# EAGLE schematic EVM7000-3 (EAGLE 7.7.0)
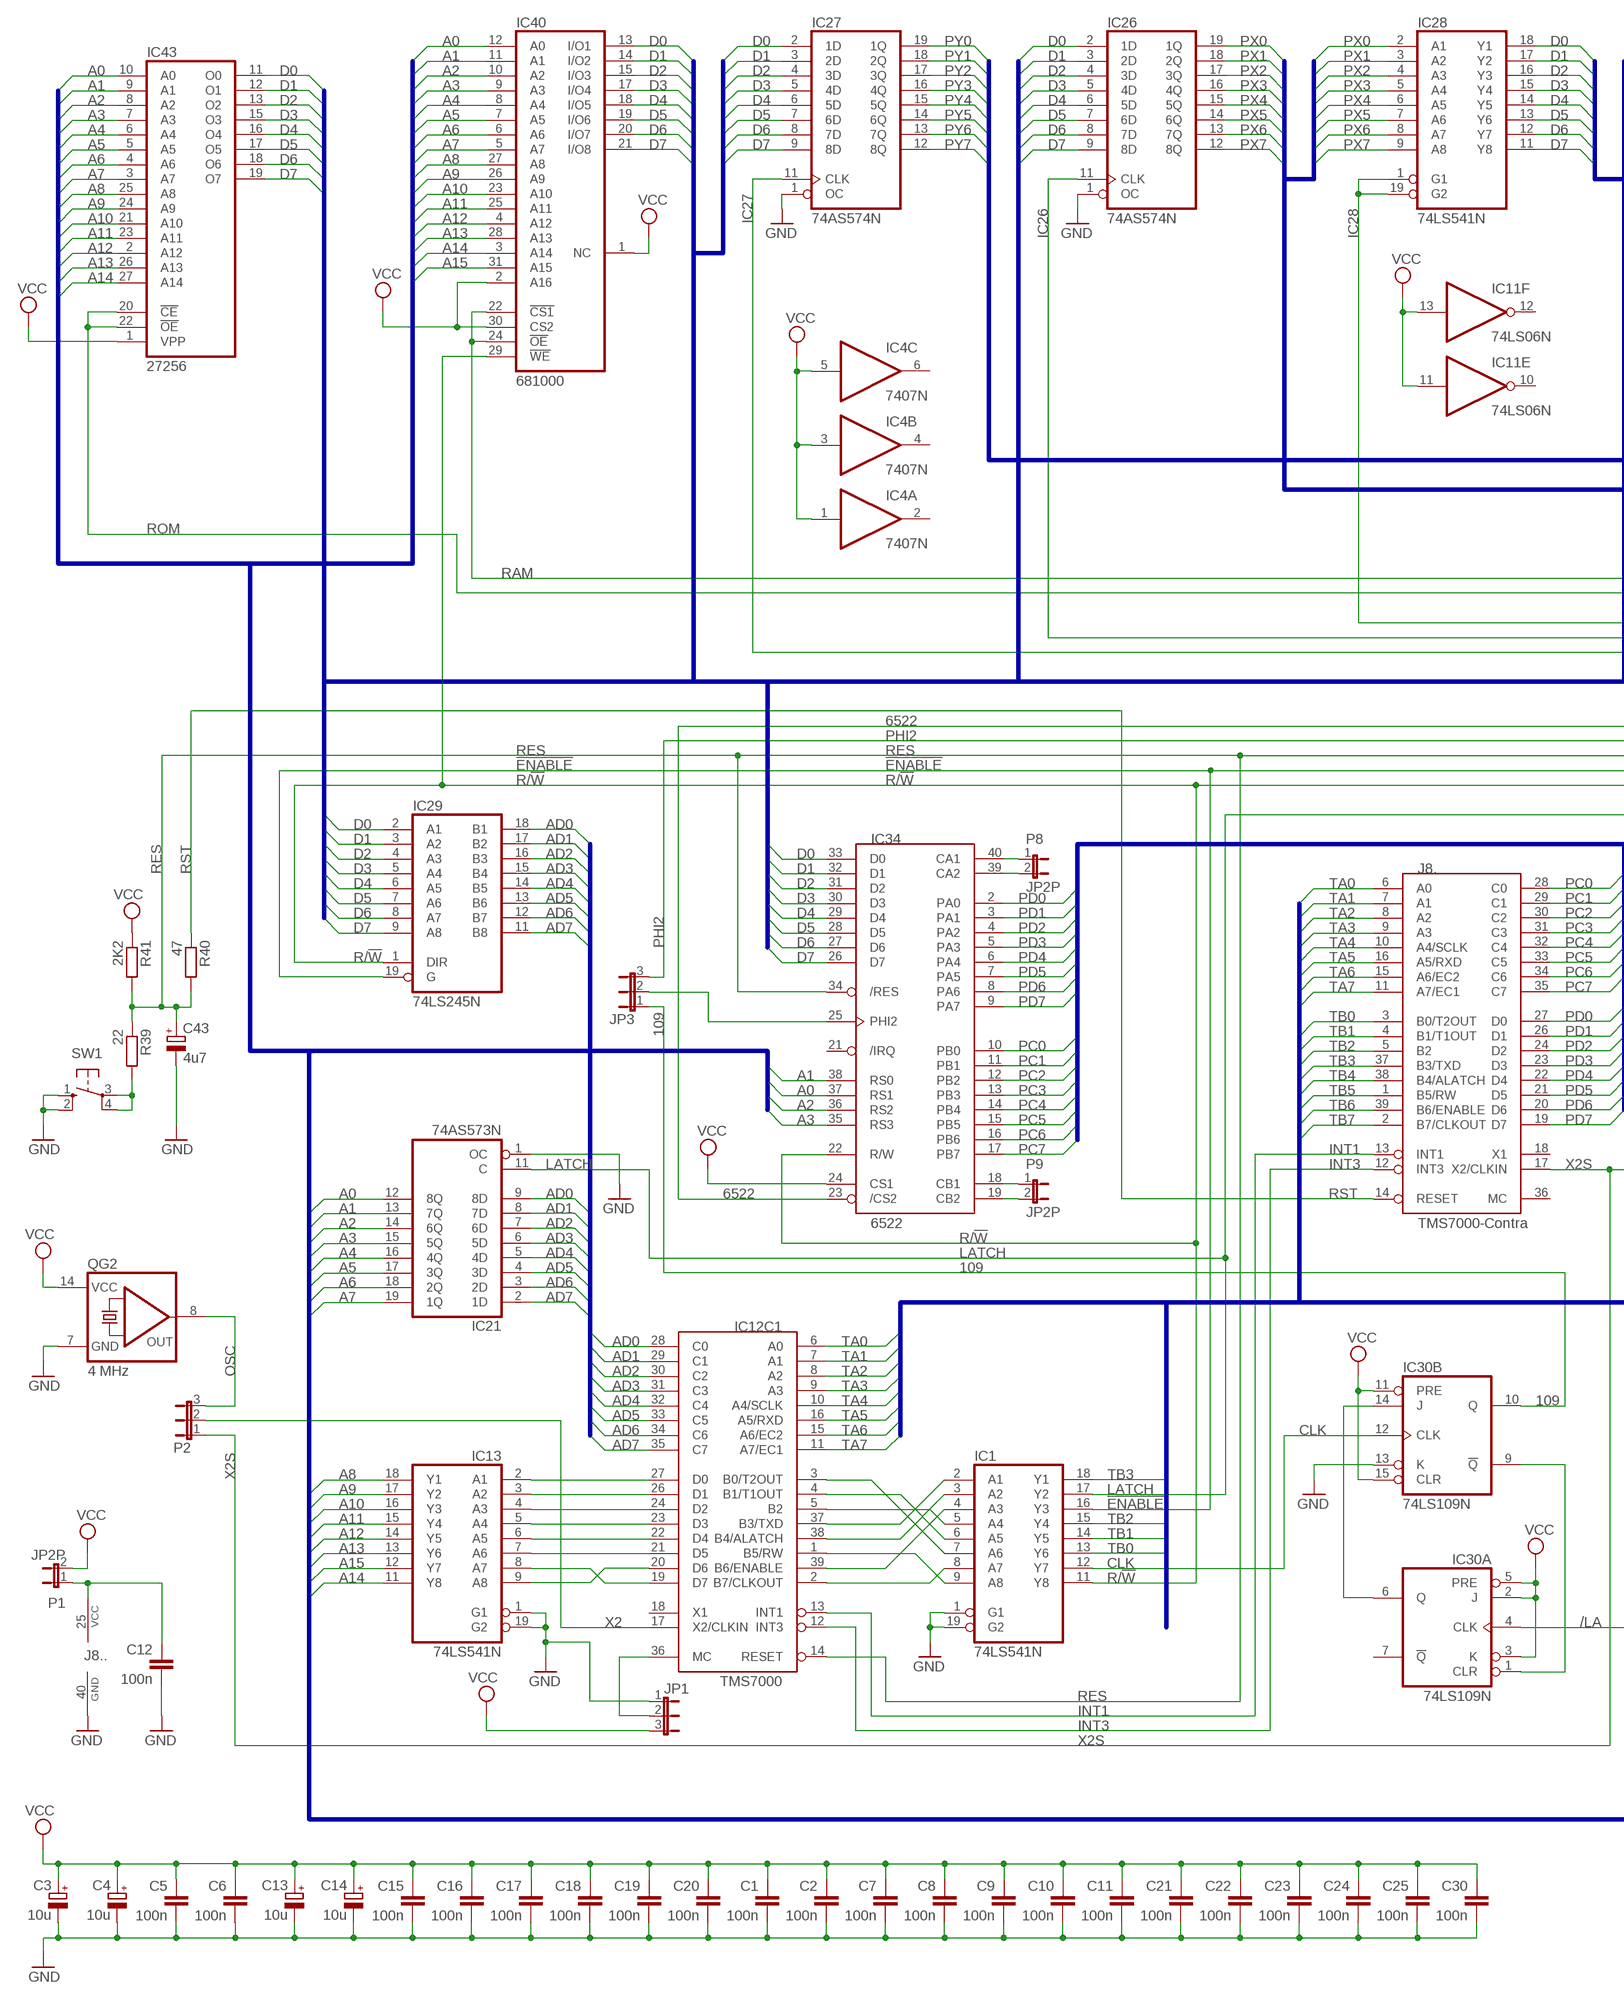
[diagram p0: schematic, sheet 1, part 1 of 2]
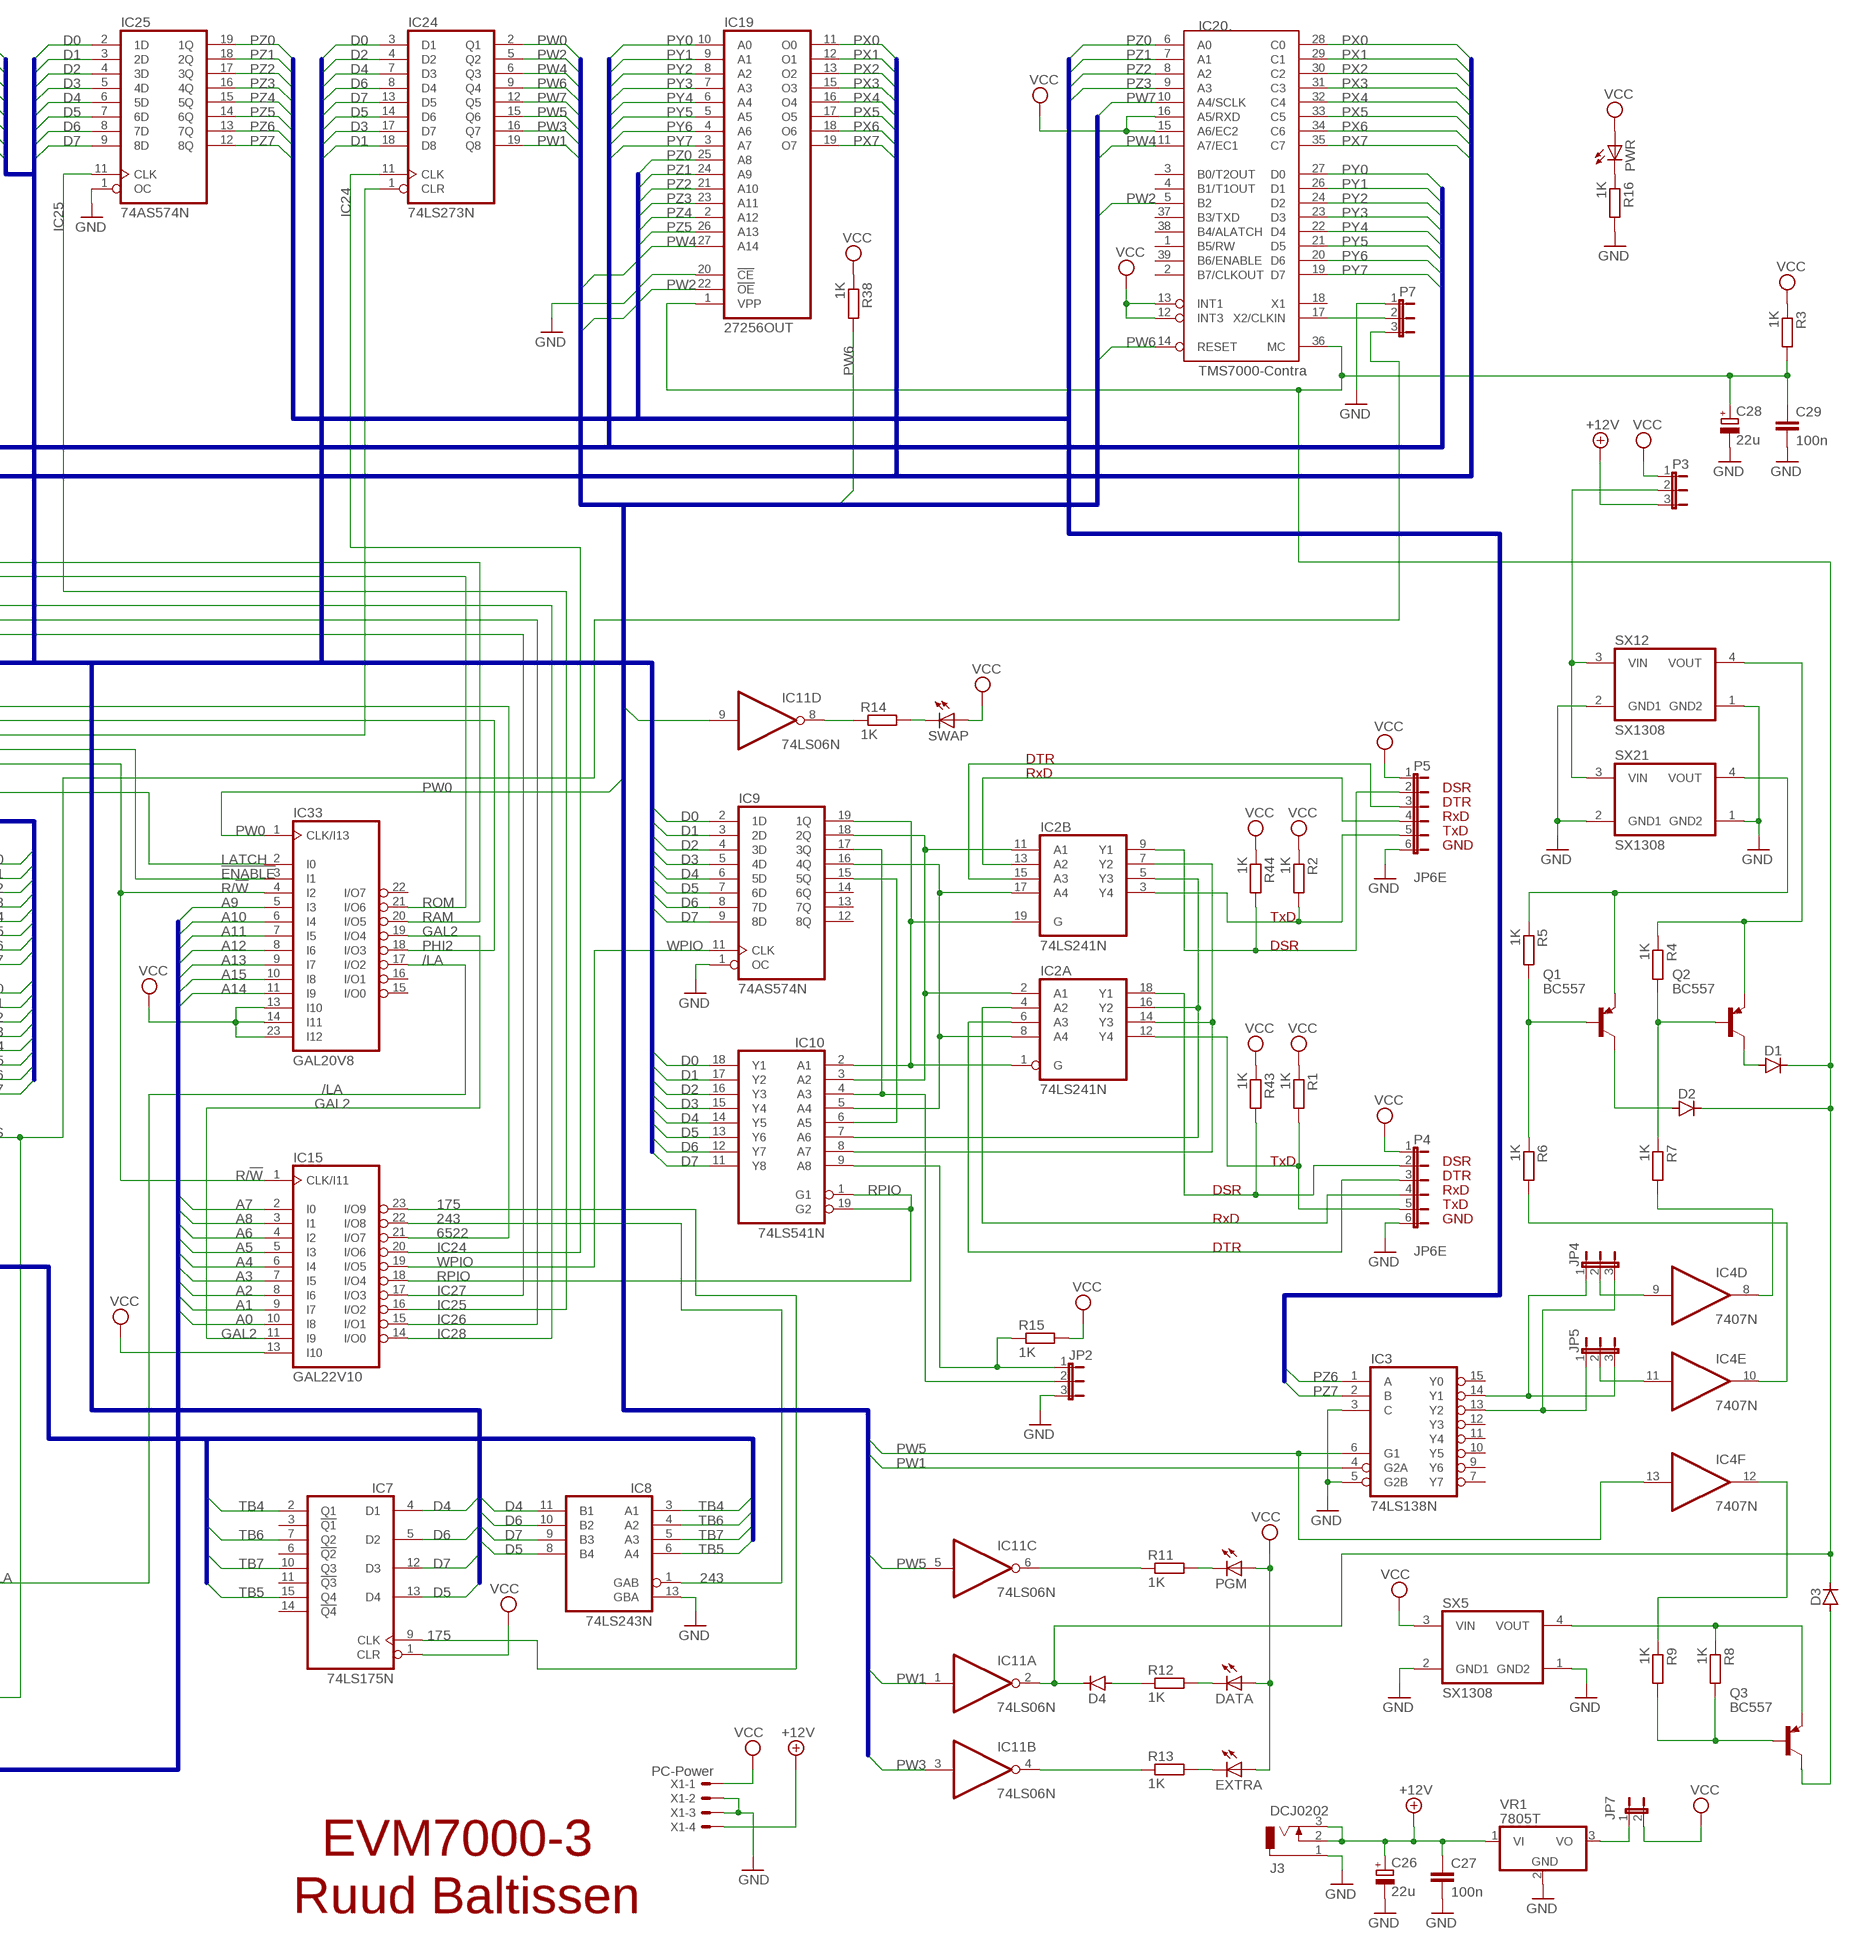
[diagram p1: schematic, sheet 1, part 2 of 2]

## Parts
C1  100n  C-EU050-024X044  [C050-024X044]
C2  100n  C-EU050-024X044  [C050-024X044]
C3  10u  CPOL-EUE5-4  [E5-4]
C4  10u  CPOL-EUE5-4  [E5-4]
C5  100n  C-EU050-024X044  [C050-024X044]
C6  100n  C-EU050-024X044  [C050-024X044]
C7  100n  C-EU050-024X044  [C050-024X044]
C8  100n  C-EU050-024X044  [C050-024X044]
C9  100n  C-EU050-024X044  [C050-024X044]
C10  100n  C-EU050-024X044  [C050-024X044]
C11  100n  C-EU050-024X044  [C050-024X044]
C12  100n  C-EU050-024X044  [C050-024X044]
C13  10u  CPOL-EUE5-4  [E5-4]
C14  10u  CPOL-EUE5-4  [E5-4]
C15  100n  C-EU050-024X044  [C050-024X044]
C16  100n  C-EU050-024X044  [C050-024X044]
C17  100n  C-EU050-024X044  [C050-024X044]
C18  100n  C-EU050-024X044  [C050-024X044]
C19  100n  C-EU050-024X044  [C050-024X044]
C20  100n  C-EU050-024X044  [C050-024X044]
C21  100n  C-EU050-024X044  [C050-024X044]
C22  100n  C-EU050-024X044  [C050-024X044]
C23  100n  C-EU050-024X044  [C050-024X044]
C24  100n  C-EU050-024X044  [C050-024X044]
C25  100n  C-EU050-024X044  [C050-024X044]
C26  22u  CPOL-EUE2,5-6E  [E2,5-6E]
C27  100n  C-EU050-024X044  [C050-024X044]
C28  22u  CPOL-EUE2,5-6E  [E2,5-6E]
C29  100n  C-EU050-024X044  [C050-024X044]
C30  100n  C-EU050-024X044  [C050-024X044]
C43  4u7  CPOL-EUE5-4  [E5-4]
D1  DIODE-S2  [0207/2V]
D2  DIODE-S2  [0207/2V]
D3  DIODE-S2  [0207/2V]
D4  DIODE-S2  [0207/2V]
DATA  TLLY4400  [LED3MM]
EXTRA  TLLY4400  [LED3MM]
IC1  74LS541N  [DIL20]
IC2  74LS241N  [DIL20]
IC3  74LS138N  [DIL16]
IC4  7407N  [DIL14]
IC7  74LS175N  [DIL16]
IC8  74LS243N  [DIL14]
IC9  74AS574N  [DIL20]
IC10  74LS541N  [DIL20]
IC11  74LS06N  [DIL14]
IC12  TMS7000  [DIL40]
IC13  74LS541N  [DIL20]
IC15  GAL22V10  [DIL24-3]
IC19  27256OUT  [DIL28]
IC20  TMS7000-Contra  TMS7000CON  [DIL40]
IC21  74AS573N  [DIL20]
IC24  74LS273N  74273N  [DIL20]
IC25  74AS574N  [DIL20]
IC26  74AS574N  [DIL20]
IC27  74AS574N  [DIL20]
IC28  74LS541N  [DIL20]
IC29  74LS245N  [DIL20]
IC30  74LS109N  [DIL16]
IC33  GAL20V8  [DIL24-3]
IC34  6522  [DIP40]
IC40  681000  [DIL32-6]
IC43  27256  [DIL28]
J3  DCJ0202  [DCJ0202]
J8  TMS7000-Contra  TMS7000CON  [DIL40]
JP1  JP2E  [JP2]
JP2  JP2E  [JP2]
JP3  JP2E  [JP2]
JP4  JP2E  [JP2]
JP5  JP2E  [JP2]
JP7  JP2P  [JP2P]
P1  JP2P  [JP2P]
P2  JP2E  [JP2]
P3  JP2E  [JP2]
P4  JP6E  [JP6E]
P5  JP6E  [JP6E]
P7  JP2E  [JP2]
P8  JP2P  [JP2P]
P9  JP2P  [JP2P]
PGM  TLLY4400  [LED3MM]
PWR  TLLY4400  [LED3MM]
Q1  BC557  [TO92-EBC]
Q2  BC557  [TO92-EBC]
Q3  BC557  [TO92-EBC]
QG2  4 MHz  QG5860  [DIL14S]
R1  1K  R-EU_0204/2V  [0204V]
R2  1K  R-EU_0204/2V  [0204V]
R3  1K  R-EU_0204/2V  [0204V]
R4  1K  R-EU_0204/2V  [0204V]
R5  1K  R-EU_0204/2V  [0204V]
R6  1K  R-EU_0204/2V  [0204V]
R7  1K  R-EU_0204/2V  [0204V]
R8  1K  R-EU_0204/2V  [0204V]
R9  1K  R-EU_0204/2V  [0204V]
R11  1K  R-EU_0204/2V  [0204V]
R12  1K  R-EU_0204/2V  [0204V]
R13  1K  R-EU_0204/2V  [0204V]
R14  1K  R-EU_0204/2V  [0204V]
R15  1K  R-EU_0204/2V  [0204V]
R16  1K  R-EU_0204/2V  [0204V]
R38  1K  R-EU_0204/2V  [0204V]
R39  22  R-EU_0204/2V  [0204V]
R40  47  R-EU_0204/2V  [0204V]
R41  2K2  R-EU_0204/2V  [0204V]
R43  1K  R-EU_0204/2V  [0204V]
R44  1K  R-EU_0204/2V  [0204V]
SW1  10-XX  [B3F-10XX]
SWAP  TLLY4400  [LED3MM]
SX5  SX1308  [SX1308]
SX12  SX1308  [SX1308]
SX21  SX1308  [SX1308]
VR1  7805T  [TO220H]
X1  PC-Power  22-23-2041  [22-23-2041]

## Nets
109: IC30.10(B:Q) JP3.1
175: IC7.9(CLK) IC15.23(I/O9)
243: IC8.1(GAB) IC15.22(I/O8)
6522: IC15.21(I/O7) IC34.23(/CS2)
!ENABLE: IC1.16(Y3) IC29.19(G) IC33.3(I1)
+12V: C26.+ C27.1 J3.2 J3.3 P3.3 VR1.1(VI) X1.4
/LA: IC30.4(A:CLK) IC33.17(I/O2)
A0: IC15.10(I8) IC21.12(8Q) IC34.37(RS1) IC40.12(A0) IC43.10(A0)
A1: IC15.9(I7) IC21.13(7Q) IC34.38(RS0) IC40.11(A1) IC43.9(A1)
A2: IC15.8(I6) IC21.14(6Q) IC34.36(RS2) IC40.10(A2) IC43.8(A2)
A3: IC15.7(I5) IC21.15(5Q) IC34.35(RS3) IC40.9(A3) IC43.7(A3)
A4: IC15.6(I4) IC21.16(4Q) IC40.8(A4) IC43.6(A4)
A5: IC15.5(I3) IC21.17(3Q) IC40.7(A5) IC43.5(A5)
A6: IC15.4(I2) IC21.18(2Q) IC40.6(A6) IC43.4(A6)
A7: IC15.2(I0) IC21.19(1Q) IC40.5(A7) IC43.3(A7)
A8: IC13.18(Y1) IC15.3(I1) IC40.27(A8) IC43.25(A8)
A9: IC13.17(Y2) IC33.5(I3) IC40.26(A9) IC43.24(A9)
A10: IC13.16(Y3) IC33.6(I4) IC40.23(A10) IC43.21(A10)
A11: IC13.15(Y4) IC33.7(I5) IC40.25(A11) IC43.23(A11)
A12: IC13.14(Y5) IC33.8(I6) IC40.4(A12) IC43.2(A12)
A13: IC13.13(Y6) IC33.9(I7) IC40.28(A13) IC43.26(A13)
A14: IC13.11(Y8) IC33.11(I9) IC40.3(A14) IC43.27(A14)
A15: IC13.12(Y7) IC33.10(I8) IC40.31(A15)
AD0: IC12.28(C1:C0) IC21.9(8D) IC29.18(B1)
AD1: IC12.29(C1:C1) IC21.8(7D) IC29.17(B2)
AD2: IC12.30(C1:C2) IC21.7(6D) IC29.16(B3)
AD3: IC12.31(C1:C3) IC21.6(5D) IC29.15(B4)
AD4: IC12.32(C1:C4) IC21.5(4D) IC29.14(B5)
AD5: IC12.33(C1:C5) IC21.4(3D) IC29.13(B6)
AD6: IC12.34(C1:C6) IC21.3(2D) IC29.12(B7)
AD7: IC12.35(C1:C7) IC21.2(1D) IC29.11(B8)
CLK: IC1.12(Y7) IC30.12(B:CLK)
D0: IC9.2(1D) IC10.18(Y1) IC24.3(D1) IC25.2(1D) IC26.2(1D) IC27.2(1D) IC28.18(Y1) IC29.2(A1) IC34.33(D0) IC40.13(I/O1) IC43.11(O0)
D1: IC9.3(2D) IC10.17(Y2) IC24.18(D8) IC25.3(2D) IC26.3(2D) IC27.3(2D) IC28.17(Y2) IC29.3(A2) IC34.32(D1) IC40.14(I/O2) IC43.12(O1)
D2: IC9.4(3D) IC10.16(Y3) IC24.4(D2) IC25.4(3D) IC26.4(3D) IC27.4(3D) IC28.16(Y3) IC29.4(A3) IC34.31(D2) IC40.15(I/O3) IC43.13(O2)
D3: IC9.5(4D) IC10.15(Y4) IC24.17(D7) IC25.5(4D) IC26.5(4D) IC27.5(4D) IC28.15(Y4) IC29.5(A4) IC34.30(D3) IC40.17(I/O4) IC43.15(O3)
D4: IC7.4(D1) IC8.11(B1) IC9.6(5D) IC10.14(Y5) IC24.7(D3) IC25.6(5D) IC26.6(5D) IC27.6(5D) IC28.14(Y5) IC29.6(A5) IC34.29(D4) IC40.18(I/O5) IC43.16(O4)
D5: IC7.13(D4) IC8.8(B4) IC9.7(6D) IC10.13(Y6) IC24.14(D6) IC25.7(6D) IC26.7(6D) IC27.7(6D) IC28.13(Y6) IC29.7(A6) IC34.28(D5) IC40.19(I/O6) IC43.17(O5)
D6: IC7.5(D2) IC8.10(B2) IC9.8(7D) IC10.12(Y7) IC24.8(D4) IC25.8(7D) IC26.8(7D) IC27.8(7D) IC28.12(Y7) IC29.8(A7) IC34.27(D6) IC40.20(I/O7) IC43.18(O6)
D7: IC7.12(D3) IC8.9(B3) IC9.9(8D) IC10.11(Y8) IC24.13(D5) IC25.9(8D) IC26.9(8D) IC27.9(8D) IC28.11(Y8) IC29.9(A8) IC34.26(D7) IC40.21(I/O8) IC43.19(O7)
DSR1: IC2.9(B:Y1) P5.2 R44.2
DSR2: IC2.18(A:Y1) P4.2 R43.2
DTR1: IC2.15(B:A3) P5.3
DTR2: IC2.6(A:A3) P4.3
GAL2: IC15.11(I9) IC33.19(I/O4)
GND: C1.2 C2.2 C3.- C4.- C5.2 C6.2 C7.2 C8.2 C9.2 C10.2 C11.2 C12.2 C13.- C14.- C15.2 C16.2 C17.2 C18.2 C19.2 C20.2 C21.2 C22.2 C23.2 C24.2 C25.2 C26.- C27.2 C28.- C29.2 C30.2 C43.- IC1.1(G1) IC1.19(G2) IC3.3(C) IC3.5(G2B) IC8.13(GBA) IC9.1(OC) IC13.1(G1) IC13.19(G2) IC19.20(!CE) IC21.1(OC) IC25.1(OC) IC26.1(OC) IC27.1(OC) IC30.13(B:K) J3.1 J8.40(..:GND) JP1.1 JP2.3 P4.6 P5.6 P7.1 QG2.7(GND) R16.2 SW1.1(S) SW1.2(S1) SX5.1(GND2) SX5.2(GND1) SX12.1(GND2) SX12.2(GND1) SX21.1(GND2) SX21.2(GND1) VR1.2(GND) X1.2 X1.3
IC24: IC15.20(I/O6) IC24.11(CLK)
IC25: IC15.16(I/O2) IC25.11(CLK)
IC26: IC15.15(I/O1) IC26.11(CLK)
IC27: IC15.17(I/O3) IC27.11(CLK)
IC28: IC15.14(I/O0) IC28.1(G1) IC28.19(G2)
INT1: IC12.13(C1:INT1) J8.13(.:INT1)
INT3: IC12.12(C1:INT3) J8.12(.:INT3)
LATCH: IC1.17(Y2) IC21.11(C) IC33.2(I0)
N$1: IC1.9(A8) IC12.1(C1:B5/RW)
N$2: IC1.8(A7) IC12.2(C1:B7/CLKOUT)
N$3: IC1.7(A6) IC12.3(C1:B0/T2OUT)
N$4: R39.2 SW1.3(P) SW1.4(P1)
N$5: IC1.6(A5) IC12.4(C1:B1/T1OUT)
N$6: IC12.19(C1:D7) IC13.8(A7)
N$7: IC12.20(C1:D6) IC13.9(A8)
N$8: IC1.5(A4) IC12.5(C1:B2)
N$9: IC1.4(A3) IC12.39(C1:B6/ENABLE)
N$10: IC12.27(C1:D0) IC13.2(A1)
N$11: IC12.26(C1:D1) IC13.3(A2)
N$12: IC12.24(C1:D2) IC13.4(A3)
N$13: IC1.3(A2) IC12.38(C1:B4/ALATCH)
N$14: C12.1 J8.25(..:VCC) P1.1
N$15: IC1.2(A1) IC12.37(C1:B3/TXD)
N$16: EXTRA.K(C) R13.2
N$17: IC12.23(C1:D3) IC13.5(A4)
N$18: IC12.22(C1:D4) IC13.6(A5)
N$19: IC12.21(C1:D5) IC13.7(A6)
N$20: IC11.4(B:O) R13.1
N$21: IC34.40(CA1) P8.1
N$22: IC34.39(CA2) P8.2
N$23: IC20.17(.:X2/CLKIN) P7.2
N$24: IC34.18(CB1) P9.1
N$25: IC34.19(CB2) P9.2
N$26: IC2.8(A:A4) IC2.17(B:A4) IC9.16(4Q) IC10.5(A4)
N$27: IC2.2(A:A1) IC2.11(B:A1) IC9.18(2Q) IC10.3(A2)
N$28: IC2.5(B:Y3) IC2.16(A:Y2) IC10.7(A6)
N$29: IC2.7(B:Y2) IC2.14(A:Y3) IC10.8(A7)
N$30: IC2.1(A:G) IC2.19(B:G) IC9.19(1Q) IC10.2(A1)
N$31: IC9.17(3Q) IC10.4(A3) JP2.2
N$32: IC9.15(5Q) IC10.6(A5)
N$33: IC4.9(D:I) JP4.2
N$34: IC4.11(E:I) JP5.2
N$36: Q1.E R5.1 SX21.4(VOUT)
N$37: Q2.E R4.1 SX12.4(VOUT)
N$38: Q1.B R5.2 R6.1
N$39: IC4.8(D:O) R7.2
N$40: Q2.B R4.2 R7.1
N$41: C28.+ C29.1 D1.2(C) D2.2(C) D3.2(C) D4.2(C) IC11.2(A:O) IC19.1(VPP) IC20.36(.:MC) R3.2
N$42: IC4.10(E:O) R6.2
N$43: Q3.B R8.2 R9.2
N$44: D1.1(A) Q2.C
N$45: IC4.12(F:O) R9.1
N$46: IC10.9(A8) JP2.1 R15.1
N$47: D2.1(A) Q1.C
N$48: D3.1(A) Q3.C
N$49: Q3.E R8.1 SX5.4(VOUT)
N$50: R14.2 SWAP.K(C)
N$51: P3.2 SX12.3(VIN) SX21.3(VIN)
N$52: IC11.8(D:O) R14.1
N$53: PWR.K(C) R16.1
N$54: IC3.14(Y1) JP4.1 JP5.3
N$55: IC3.13(Y2) JP4.3 JP5.1
N$56: PGM.K(C) R11.2
N$57: DATA.K(C) R12.2
N$58: D4.1(A) R12.1
N$59: IC12.36(C1:MC) JP1.2
N$60: IC11.6(C:O) R11.1
N$63: IC34.25(PHI2) JP3.2
N$64: IC30.6(A:Q) IC30.14(B:J)
N$65: JP7.1 VR1.3(VO)
N$66: IC30.1(A:CLR) IC30.9(B:!Q)
OSC: P2.3 QG2.8(OUT)
PC0: IC34.10(PB0) J8.28(.:C0)
PC1: IC34.11(PB1) J8.29(.:C1)
PC2: IC34.12(PB2) J8.30(.:C2)
PC3: IC34.13(PB3) J8.31(.:C3)
PC4: IC34.14(PB4) J8.32(.:C4)
PC5: IC34.15(PB5) J8.33(.:C5)
PC6: IC34.16(PB6) J8.34(.:C6)
PC7: IC34.17(PB7) J8.35(.:C7)
PD0: IC34.2(PA0) J8.27(.:D0)
PD1: IC34.3(PA1) J8.26(.:D1)
PD2: IC34.4(PA2) J8.24(.:D2)
PD3: IC34.5(PA3) J8.23(.:D3)
PD4: IC34.6(PA4) J8.22(.:D4)
PD5: IC34.7(PA5) J8.21(.:D5)
PD6: IC34.8(PA6) J8.20(.:D6)
PD7: IC34.9(PA7) J8.19(.:D7)
PHI2: IC33.18(I/O3) JP3.3
PW0: IC11.9(D:I) IC24.2(Q1) IC33.1(CLK/I13)
PW1: IC3.4(G2A) IC11.1(A:I) IC24.19(Q8)
PW2: IC19.22(!OE) IC20.5(.:B2) IC24.5(Q2)
PW3: IC11.3(B:I) IC24.16(Q7)
PW4: IC19.27(A14) IC20.11(.:A7/EC1) IC24.6(Q3)
PW5: IC3.6(G1) IC4.13(F:I) IC11.5(C:I) IC24.15(Q6)
PW6: IC20.14(.:RESET) IC24.9(Q4) R38.2
PW7: IC20.10(.:A4/SCLK) IC24.12(Q5)
PX0: IC19.11(O0) IC20.28(.:C0) IC26.19(1Q) IC28.2(A1)
PX1: IC19.12(O1) IC20.29(.:C1) IC26.18(2Q) IC28.3(A2)
PX2: IC19.13(O2) IC20.30(.:C2) IC26.17(3Q) IC28.4(A3)
PX3: IC19.15(O3) IC20.31(.:C3) IC26.16(4Q) IC28.5(A4)
PX4: IC19.16(O4) IC20.32(.:C4) IC26.15(5Q) IC28.6(A5)
PX5: IC19.17(O5) IC20.33(.:C5) IC26.14(6Q) IC28.7(A6)
PX6: IC19.18(O6) IC20.34(.:C6) IC26.13(7Q) IC28.8(A7)
PX7: IC19.19(O7) IC20.35(.:C7) IC26.12(8Q) IC28.9(A8)
PY0: IC19.10(A0) IC20.27(.:D0) IC27.19(1Q)
PY1: IC19.9(A1) IC20.26(.:D1) IC27.18(2Q)
PY2: IC19.8(A2) IC20.24(.:D2) IC27.17(3Q)
PY3: IC19.7(A3) IC20.23(.:D3) IC27.16(4Q)
PY4: IC19.6(A4) IC20.22(.:D4) IC27.15(5Q)
PY5: IC19.5(A5) IC20.21(.:D5) IC27.14(6Q)
PY6: IC19.4(A6) IC20.20(.:D6) IC27.13(7Q)
PY7: IC19.3(A7) IC20.19(.:D7) IC27.12(8Q)
PZ0: IC19.25(A8) IC20.6(.:A0) IC25.19(1Q)
PZ1: IC19.24(A9) IC20.7(.:A1) IC25.18(2Q)
PZ2: IC19.21(A10) IC20.8(.:A2) IC25.17(3Q)
PZ3: IC19.23(A11) IC20.9(.:A3) IC25.16(4Q)
PZ4: IC19.2(A12) IC25.15(5Q)
PZ5: IC19.26(A13) IC25.14(6Q)
PZ6: IC3.1(A) IC25.13(7Q)
PZ7: IC3.2(B) IC25.12(8Q)
R/!W: IC1.11(Y8) IC15.1(CLK/I11) IC29.1(DIR) IC33.4(I2) IC34.22(R/W) IC40.29(!WE)
RAM: IC33.20(I/O5) IC40.22(!CS1) IC40.24(!OE)
RES: C43.+ IC12.14(C1:RESET) IC24.1(CLR) IC34.34(/RES) R39.1 R40.2 R41.2
ROM: IC33.21(I/O6) IC43.20(!CE) IC43.22(!OE)
RPIO: IC10.1(G1) IC10.19(G2) IC15.18(I/O4)
RST: J8.14(.:RESET) R40.1
RXD1: IC2.13(B:A2) P5.4
RXD2: IC2.4(A:A2) P4.4
TA0: IC12.6(C1:A0) J8.6(.:A0)
TA1: IC12.7(C1:A1) J8.7(.:A1)
TA2: IC12.8(C1:A2) J8.8(.:A2)
TA3: IC12.9(C1:A3) J8.9(.:A3)
TA4: IC12.10(C1:A4/SCLK) J8.10(.:A4/SCLK)
TA5: IC12.16(C1:A5/RXD) J8.16(.:A5/RXD)
TA6: IC12.15(C1:A6/EC2) J8.15(.:A6/EC2)
TA7: IC12.11(C1:A7/EC1) J8.11(.:A7/EC1)
TB0: IC1.13(Y6) J8.3(.:B0/T2OUT)
TB1: IC1.14(Y5) J8.4(.:B1/T1OUT)
TB2: IC1.15(Y4) J8.5(.:B2)
TB3: IC1.18(Y1) J8.37(.:B3/TXD)
TB4: IC7.2(Q1) IC8.3(A1) J8.38(.:B4/ALATCH)
TB5: IC7.15(Q4) IC8.6(A4) J8.1(.:B5/RW)
TB6: IC7.7(Q2) IC8.4(A2) J8.39(.:B6/ENABLE)
TB7: IC7.10(Q3) IC8.5(A3) J8.2(.:B7/CLKOUT)
TXD1: IC2.3(B:Y4) P5.5 R2.2
TXD2: IC2.12(A:Y4) P4.5 R1.2
VCC: C1.1 C2.1 C3.+ C4.+ C5.1 C6.1 C7.1 C8.1 C9.1 C10.1 C11.1 C13.+ C14.+ C15.1 C16.1 C17.1 C18.1 C19.1 C20.1 C21.1 C22.1 C23.1 C24.1 C25.1 C30.1 DATA.A EXTRA.A IC4.1(A:I) IC4.3(B:I) IC4.5(C:I) IC7.1(CLR) IC11.11(E:I) IC11.13(F:I) IC15.13(I10) IC20.12(.:INT3) IC20.13(.:INT1) IC20.15(.:A6/EC2) IC20.16(.:A5/RXD) IC30.2(A:J) IC30.3(A:K) IC30.5(A:PRE) IC30.11(B:PRE) IC30.15(B:CLR) IC33.13(I10) IC33.14(I11) IC33.23(I12) IC34.24(CS1) IC40.1(NC) IC40.2(A16) IC40.30(CS2) IC43.1(VPP) JP1.3 JP7.2 P1.2 P3.1 P4.1 P5.1 PGM.A PWR.A QG2.14(VCC) R1.1 R2.1 R3.1 R15.2 R38.1 R41.1 R43.1 R44.1 SWAP.A SX5.3(VIN) X1.1
WPIO: IC9.11(CLK) IC15.19(I/O5)
X2: IC12.17(C1:X2/CLKIN) P2.2
X2S: J8.17(.:X2/CLKIN) P2.1 P7.3
Unconnected: IC3.7(Y7) IC3.9(Y6) IC3.10(Y5) IC3.11(Y4) IC3.12(Y3) IC3.15(Y0) IC4.2(A:O) IC4.4(B:O) IC4.6(C:O) IC7.3(!Q1) IC7.6(!Q2) IC7.11(!Q3) IC7.14(!Q4) IC9.12(8Q) IC9.13(7Q) IC9.14(6Q) IC11.10(E:O) IC11.12(F:O) IC12.18(C1:X1) IC20.1(.:B5/RW) IC20.2(.:B7/CLKOUT) IC20.3(.:B0/T2OUT) IC20.4(.:B1/T1OUT) IC20.18(.:X1) IC20.37(.:B3/TXD) IC20.38(.:B4/ALATCH) IC20.39(.:B6/ENABLE) IC30.7(A:!Q) IC33.15(I/O0) IC33.16(I/O1) IC33.22(I/O7) IC34.21(/IRQ) J8.18(.:X1) J8.36(.:MC)

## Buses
ADDRESSBUS:A[0..15]
DATABUS:D[0..7]
ADDA:AD[0..7]
TMS:TA[0..7],TB[0..7]
PCD:PC[0..7],PD[0..7]
PY:PY[0..7]
PX:PX[0..7]
PZ:PZ[0..7]
PW:PW[0..7]

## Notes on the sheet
- DTR
- RxD
- DSR
- DTR
- RxD
- TxD
- GND
- TxD
- DSR
- TxD | DSR
- DTR
- DSR | RxD
- TxD
- RxD | GND
- DTR
- EVM7000-3
- Ruud Baltissen

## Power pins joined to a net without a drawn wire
GND: IC1.10(GND) IC2.10(P:GND) IC3.8(GND) IC4.7(P:GND) IC7.8(GND) IC8.7(GND) IC9.10(GND) IC10.10(GND) IC11.7(P:GND) IC12.40(GND) IC13.10(GND) IC15.12(GND) IC19.14(GND) IC20.40(..:GND) IC21.10(GND) IC24.10(GND) IC25.10(GND) IC26.10(GND) IC27.10(GND) IC28.10(GND) IC29.10(GND) IC30.8(P:GND) IC33.12(GND) IC34.1(GND) IC40.16(GND) IC43.14(GND)
VCC: IC1.20(VCC) IC2.20(P:VCC) IC3.16(VCC) IC4.14(P:VCC) IC7.16(VCC) IC8.14(VCC) IC9.20(VCC) IC10.20(VCC) IC11.14(P:VCC) IC12.25(VCC) IC13.20(VCC) IC15.24(VCC) IC19.28(VCC) IC20.25(..:VCC) IC21.20(VCC) IC24.20(VCC) IC25.20(VCC) IC26.20(VCC) IC27.20(VCC) IC28.20(VCC) IC29.20(VCC) IC30.16(P:VCC) IC33.24(VCC) IC34.20(VCC) IC40.32(VCC) IC43.28(VCC)

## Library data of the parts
C1 C2 C5-C12 C15-C25 C27 C29 C30 = rcl:C-EU: CAPACITOR, European symbol
C3 C4 C13 C14 C43 = resistor:CPOL-EU: POLARIZED CAPACITOR, European symbol
C26 C28 = rcl:CPOL-EU: POLARIZED CAPACITOR, European symbol
D1-D4 = 0RB_Passive:DIODE-S2: DIODE
DATA EXTRA PGM PWR SWAP = led:TLLY4400: Low Current (2mA) LED 3 mm Tinted Diffused Package color YELLOW; MF: VISHAY SEMICONDUCTOR; OC_FARNELL: 1612439
IC1 IC10 IC13 IC28 = 74xx-us:74*541: Octal BUFFER and LINE DRIVER, 3-state
IC2 = 74xx-us:74*241: Octal BUFFER and LINE DRIVER, 3-state
IC3 = 0RB_TTL:74*138: 3-line to 8-line DECODER/DEMULTIPLEXER smaller then original version
IC4 = 74xx-us:74*07: Hex BUFFER, open collector high-voltage output
IC7 = 74xx-us:74*175: Qadruple D type FLIP FLOP, clear
IC8 = 74xx-us:74*243: Quadruple BUS TRANSCEIVER
IC9 IC25-IC27 = 74xx-us:74*574: 8-bit D type FLIP FLOP bus driver
IC11 = 74xx-us:74*06: Hex INVERTER, open collector high-voltage output
IC12 = 0RB_CPU:TMS7000
IC15 = 0RB_GAL:GAL22V10: GAL; MPN: GAL22V10D-7LPN; OC_FARNELL: 1571925; OC_NEWARK: 97M0480
IC19 = 0RB_Memory:27256OUT: 27256 counterpart. Enables user to replace the EPROM with a PCB.
IC20 J8 = 0RB_CPU:TMS7000CON
IC21 = 74xx-us:74*573: 8-bit D latch BUS DRIVER
IC24 = 74xx-us:74*273: Octal D type FLIP FLOP, clear
IC29 = 74xx-us:74*245: Octal BUS TRANSCEIVER, 3-state
IC30 = 74xx-us:74*109: Dual J-K positive edge triggered FLIP FLOP, preset and clear
IC33 = 0RB_GAL:GAL20V8: GAL; MPN: GAL22V10D-7LPN; OC_FARNELL: 1571925; OC_NEWARK: 97M0480
IC34 = 0RB_65xx:6522: I/O device: two 8-bits ports, handshake lines, timers.
IC40 = 0RB_Memory:681000: 128K*8 SRAM
IC43 = 0RB_Memory:27256: 32K*8 EPROM
J3 = con-jack:DCJ0202: DC POWER JACK Source: DCJ0202.pdf; OC_FARNELL: unknown; OC_NEWARK: unknown
JP1-JP5 P2 P3 P7 = jumper:JP2E: JUMPER
JP7 P1 P8 P9 = 0RB_Connectors:JP2P
P4 P5 = 0RB_Connectors:JP6E
Q1-Q3 = transistor-pnp:BC557*: PNP Transistror
QG2 = crystal:QG5860: CRYSTAL RESONATOR; OC_FARNELL: unknown; OC_NEWARK: unknown
R1-R9 R11-R16 R38-R41 R43 R44 = rcl:R-EU_: RESISTOR, European symbol
SW1 = switch-omron:10-XX: OMRON SWITCH; MPN: B3F-1000; OC_FARNELL: 176432; OC_NEWARK: 36M3542
SX5 SX12 SX21 = 0RB_Lineair:SX1308
VR1 = linear:78*: Positive VOLTAGE REGULATOR Source: http://cache.national.com/ds/LM/LM78L05.pdf http://www.fairchildsemi.com/ds/LM/LM7805.pdf
X1 = con-molex:22-23-2041: .100" (2.54mm) Center Header - 4 Pin; MF: MOLEX; MPN: 22-23-2041; OC_FARNELL: 1462920; OC_NEWARK: 38C0355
